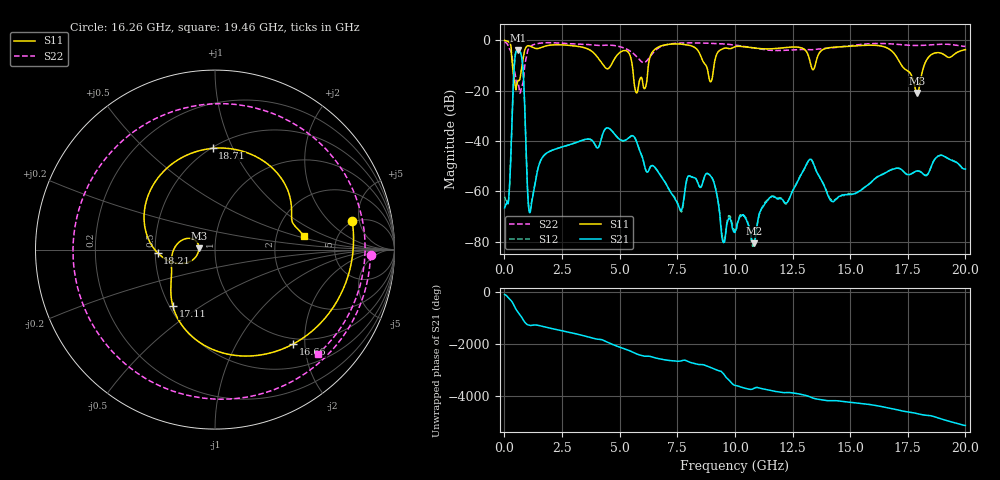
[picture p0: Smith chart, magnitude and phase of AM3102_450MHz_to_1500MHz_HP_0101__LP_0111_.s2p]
!Agilent Technologies,E8364B,MY43040894,A.07.50.67
!Agilent E8364B: A.07.50.67
!Date: Thursday, January 11, 2018 05:41:31
!Correction: S11(Full 2 Port(1,2))
!S21(Full 2 Port(1,2))
!S12(Full 2 Port(1,2))
!S22(Full 2 Port(1,2))
!S2P File: Measurements: S11, S21, S12, S22:
# Hz S  dB  R 50
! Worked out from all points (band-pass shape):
!   1601 points, 10 MHz to 20 GHz, reference 50 ohm
!   highest |S21| = -3.81 dB at 584.7 MHz (marker M1); lowest = -80.5 dB at 10.83 GHz (marker M2)
!   |S21| within 3 dB of the highest: 459.1 MHz to 754 MHz (294.8 MHz wide, 48.6 % of centre)
!   lowest |S11| = -20.9 dB at 17.9 GHz (marker M3), VSWR 1.20, Z = 41.7 + j0.609 ohm
!   |S11| at or under -10 dB: 350.5 MHz to 765.5 MHz (415 MHz wide, 74.4 % of centre); 5.549 GHz to 6.245 GHz (696.3 MHz wide, 11.8 % of centre); 17.24 GHz to 18.21 GHz (973 MHz wide, 5.49 % of centre)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
!   |S22| runs from -21.0 to -0.5 dB; largest |S21 - S12| = 0.0016
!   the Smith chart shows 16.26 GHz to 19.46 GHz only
!   S11 on the Smith chart (normalised r, x): 16.26 GHz: 4.77, +3.96; 16.66 GHz: 0.89, -1.76; 17.11 GHz: 0.52, -0.39; 18.21 GHz: 0.52, -0.02; 18.71 GHz: 0.51, +0.84; 19.46 GHz: 2.89, +0.57
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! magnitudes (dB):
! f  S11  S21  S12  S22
! 10 MHz  -0.1  -66.5  -62.1  -0.5
! 184.9 MHz  -0.6  -63.3  -63.0  -2.6
! 584.7 MHz  -16.0  -3.8  -3.8  -17.5
! 784.6 MHz  -9.0  -8.9  -8.9  -17.6
! 1.109 GHz  -2.3  -68.4  -67.6  -2.6
! 3.346 GHz  -2.7  -39.8  -39.8  -1.6
! 5.732 GHz  -20.9  -40.2  -40.2  -6.4
! 6.682 GHz  -2.7  -52.3  -52.4  -3.1
! 7.656 GHz  -1.5  -67.6  -68.0  -1.1
! 8.881 GHz  -15.1  -53.2  -53.3  -1.2
! 10.01 GHz  -2.5  -76.2  -75.6  -1.9
! 10.83 GHz  -3.1  -80.5  -81.1  -3.1
! 13.34 GHz  -11.1  -47.7  -47.7  -3.7
! 16.26 GHz  -2.1  -53.8  -53.7  -1.2
! 16.66 GHz  -3.3  -51.9  -51.9  -1.3
! 16.68 GHz  -3.4  -51.8  -51.8  -1.3
! 17.11 GHz  -8.1  -50.8  -50.8  -1.7
! 17.9 GHz  -20.9  -51.9  -51.9  -2.0
! 18.21 GHz  -9.9  -53.5  -53.3  -2.0
! 18.71 GHz  -5.0  -46.8  -46.8  -1.7
! 19.46 GHz  -6.0  -47.8  -47.7  -1.8
! 20 GHz  -3.7  -51.1  -51.0  -2.4
